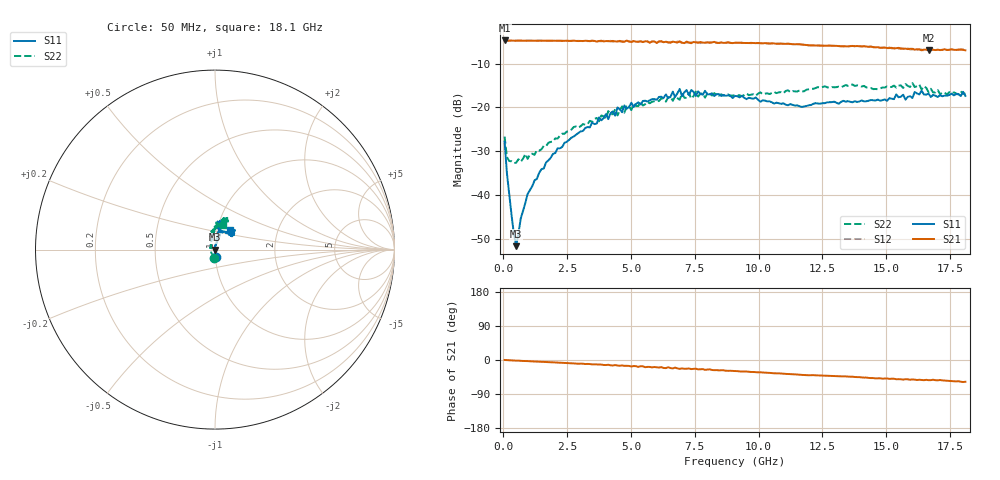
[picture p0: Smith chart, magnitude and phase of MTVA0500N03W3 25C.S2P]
! Network Analyzer HP8720D.06.14 Serial No. US36140669
!  8 Jul 2005  08:06:37
! Frequency  S11  S21  S12  S22
# HZ  S  DB R 50
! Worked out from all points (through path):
!   201 points, 50 MHz to 18.1 GHz, reference 50 ohm
!   highest |S21| = -4.74 dB at 50 MHz (marker M1); lowest = -7.0 dB at 16.66 GHz (marker M2)
!   group delay of S21, straight-line fit = 8.97 ps
!   lowest |S11| = -51.6 dB at 501.2 MHz (marker M3), VSWR 1.01, Z = 49.7 - j0.0182 ohm
!   |S11| at or under -10 dB: start of sweep to end of sweep
!   |S22| runs from -32.7 to -14.4 dB; largest |S21 - S12| = 0.023
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5e7  -27.80 -85.1  -4.74 0.1  -4.75 0.1  -26.66 -94.2
1.4025e8  -34.99 -89.9  -4.82 -0.4  -4.79 -0.4  -31.31 -138.7
5.0125e8  -51.62 -176.0  -4.80 -1.7  -4.79 -1.6  -32.62 174.7
6.8175e8  -45.32 122.9  -4.79 -2.1  -4.80 -2.1  -32.39 167.1
1.22325e9  -36.63 94.0  -4.81 -3.8  -4.81 -3.9  -30.80 142.1
2.12575e9  -29.33 78.1  -4.81 -7.0  -4.82 -6.9  -27.10 117.5
3.1185e9  -25.38 78.3  -4.86 -9.7  -4.89 -10.1  -23.81 112.1
4.382e9  -21.88 75.1  -4.96 -13.4  -4.92 -14.6  -20.39 102.2
4.47225e9  -20.01 71.6  -4.97 -14.6  -4.89 -13.7  -21.83 104.9
4.65275e9  -21.10 71.9  -5.05 -14.5  -4.87 -15.2  -19.76 103.3
4.743e9  -19.55 75.4  -5.04 -15.4  -5.01 -14.7  -21.20 99.2
6.09675e9  -17.61 75.9  -5.00 -19.8  -4.91 -19.7  -18.52 90.0
6.7285e9  -17.60 82.2  -5.12 -20.1  -5.33 -21.1  -17.46 83.9
6.909e9  -15.79 80.4  -4.94 -23.4  -5.08 -22.0  -18.26 82.6
6.99925e9  -17.44 79.9  -5.24 -22.0  -5.32 -23.8  -16.77 83.8
7.36025e9  -16.04 74.3  -5.37 -24.0  -5.16 -22.9  -18.00 88.7
9.075e9  -17.39 82.3  -5.26 -29.1  -5.24 -29.1  -17.23 78.5
1.21435e10  -19.18 66.3  -5.86 -39.9  -5.81 -40.1  -15.76 75.8
1.512175e10  -17.90 39.5  -6.48 -49.8  -6.32 -49.3  -15.39 75.6
1.602425e10  -17.87 45.7  -6.65 -51.3  -6.80 -53.2  -14.43 68.9
1.6656e10  -16.85 46.4  -7.00 -53.2  -6.93 -52.1  -16.50 65.3
1.81e10  -17.38 52.1  -7.00 -57.5  -7.16 -58.3  -16.81 73.1
